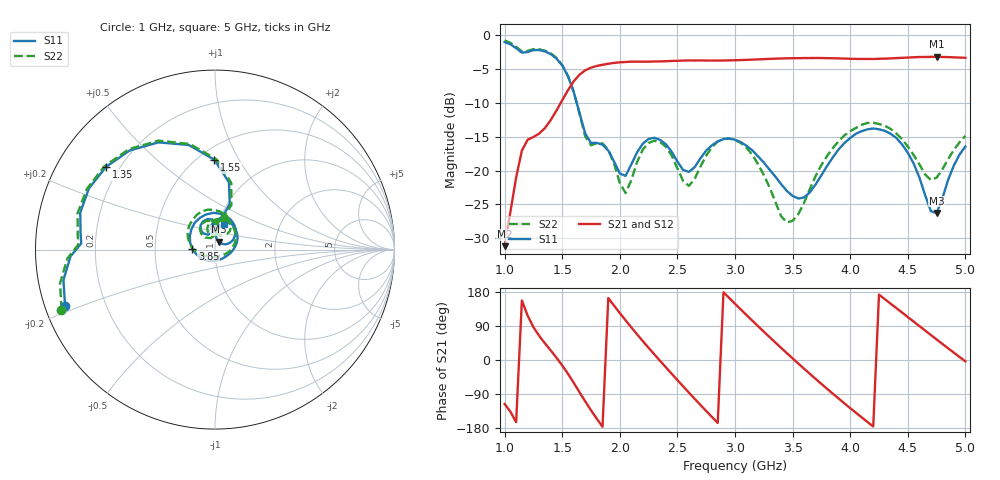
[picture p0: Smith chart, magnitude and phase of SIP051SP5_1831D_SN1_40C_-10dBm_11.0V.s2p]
# GHz  S  dB  R  50
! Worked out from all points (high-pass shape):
!   81 points, 1 GHz to 5 GHz, reference 50 ohm
!   highest |S21| = -3.16 dB at 4.75 GHz (marker M1); lowest = -31.2 dB at 1 GHz (marker M2)
!   |S21| within 3 dB of the highest: 1.632 GHz to end of sweep
!   lowest |S11| = -26.3 dB at 4.75 GHz (marker M3), VSWR 1.10, Z = 51.9 + j4.58 ohm
!   |S11| at or under -10 dB: 1.627 GHz to end of sweep
!   |S22| runs from -27.7 to -0.7 dB; largest |S21 - S12| = 0.0033
!   S11 on the Smith chart (normalised r, x): 1 GHz: 0.06, -0.18; 1.35 GHz: 0.15, +0.33; 1.55 GHz: 0.60, +0.80; 3.85 GHz: 0.78, +0.01; 5 GHz: 1.07, +0.31
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1  -0.99 -159.3  -31.18 -116.0  -31.21 -116.2  -0.74 -158.6
1.15  -2.54 177.4  -17.04 157.0  -17.05 156.8  -2.35 178.0
1.35  -2.36 142.8  -13.70 44.0  -13.71 44.0  -2.26 142.9
1.55  -6.01 90.3  -8.10 -36.5  -8.08 -36.4  -5.98 89.0
1.7  -14.53 77.0  -5.15 -109.2  -5.16 -109.2  -14.94 76.2
1.85  -16.16 93.5  -4.34 -176.1  -4.32 -176.2  -15.97 92.1
2.05  -20.79 115.4  -3.93 104.8  -3.93 104.8  -23.31 110.5
2.2  -16.00 120.5  -3.87 49.7  -3.87 49.7  -16.87 126.2
2.35  -15.46 95.1  -3.84 -2.4  -3.84 -2.4  -15.78 98.0
2.5  -18.66 80.6  -3.75 -53.1  -3.75 -52.9  -19.67 78.7
2.65  -19.48 99.4  -3.71 -102.5  -3.71 -102.4  -21.22 107.5
2.85  -15.68 83.1  -3.72 -166.0  -3.73 -166.0  -15.71 93.8
3  -15.43 55.4  -3.67 148.4  -3.66 148.4  -15.48 62.0
3.3  -19.85 -0.1  -3.47 60.5  -3.47 60.5  -22.46 -11.8
3.5  -23.75 -49.4  -3.37 4.3  -3.37 4.3  -27.43 -100.5
3.7  -22.04 -132.0  -3.34 -49.8  -3.35 -49.8  -20.79 -166.4
3.85  -18.02 178.2  -3.37 -89.1  -3.37 -89.1  -16.65 165.3
4.1  -14.16 115.1  -3.47 -151.5  -3.47 -151.5  -13.21 117.8
4.35  -14.53 61.6  -3.40 148.9  -3.41 149.0  -13.81 74.8
4.55  -18.92 27.8  -3.23 101.6  -3.24 101.6  -17.67 51.1
4.75  -26.29 65.2  -3.16 54.3  -3.18 54.2  -21.05 81.2
5  -16.43 69.5  -3.30 -3.6  -3.31 -3.5  -14.86 74.3
